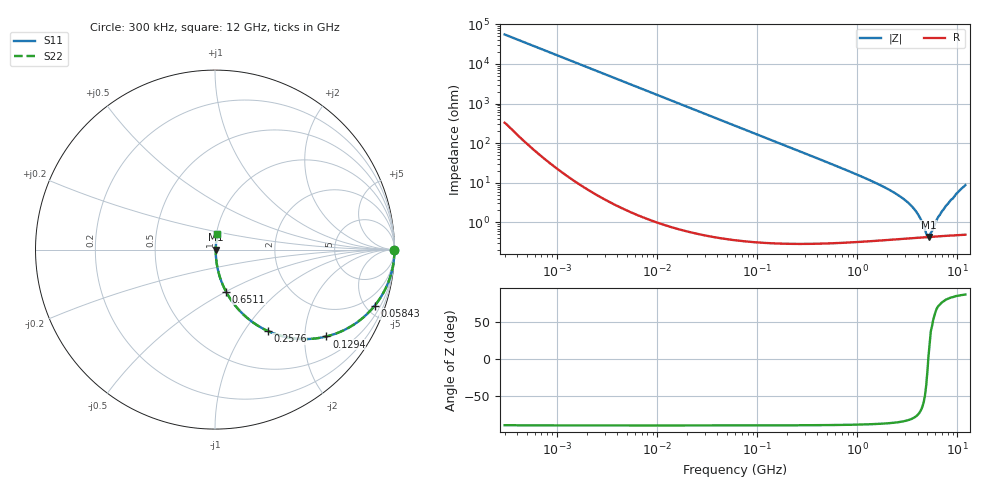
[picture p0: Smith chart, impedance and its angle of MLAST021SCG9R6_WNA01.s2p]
! MLAST021SCG9R6_WNA01  S-PARAMETER MODEL  ( General Type )
! Model Generated by TAIYO YUDEN Corporation (http://www.ty-top.com)
! Version 1.0
! TAIYO YUDEN Control No. 220901
! Copyright(c) 2022 TAIYO YUDEN CO.,LTD. All Rights Reserved.
! Product Description (link to TY-COMPAS)
! https://ds.yuden.co.jp/TYCOMPAS/or/detail?pn=MLAST021SCG9R6CWNA01&u=M
! Products Name : Multilayer Ceramic Capacitors
! Characteristics :
!  Capacitance : 9.6 pF , Rated Voltage : 25V , TCC : CG / C0G
!  Case Size : 0.25 x 0.125 / 0.0098 x 0.0049 [mm/inch] , Thickness : 0.125 / 0.0049 [mm/inch]
!  (Conditions: Temperature = 25 degC , DC Bias Current/Voltage = 0A / 0V)
! External Node Assignments :
!  1  o---| |---o  2
! GND o---------o GND
! Frequency Range : 0.3MHz  -  12000MHz  [ 401 STEP ]
# MHz S RI R 50
! Freq[MHz].  S11 Real  S11 Imag  S21 Real  S21 Imag  S12 Real  S12 Imag  S22 Real  S22 Imag
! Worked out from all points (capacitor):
!   401 points, 300 kHz to 12 GHz, reference 50 ohm
!   read as one part in series: C = 9.6 pF near 316.3 kHz
!   lowest |Z| = 428 mohm at 5.141 GHz (marker M1)
!   series resonance near 5.116 GHz, so ESL is about 100 pH
!   S11 on the Smith chart (normalised r, x): 300 kHz: open; 58.43 MHz: 1.01, -5.67; 129.4 MHz: 1.01, -2.56; 257.6 MHz: 1.01, -1.28; 651.1 MHz: 1.01, -0.50; 12 GHz: 1.01, +0.17
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0.3  1 -0.00181  1.4e-05 0.00181  1.4e-05 0.00181  1 -0.00181
1.769972  0.9999 -0.0107  0.000123 0.0107  0.000123 0.0107  0.9999 -0.0107
10.44266  0.996 -0.0627  0.00399 0.0627  0.00399 0.0627  0.996 -0.0627
25.70316  0.9764 -0.1514  0.0236 0.1514  0.0236 0.1514  0.9764 -0.1514
58.43137  0.8892 -0.3133  0.1108 0.3133  0.1108 0.3133  0.8892 -0.3133
60  0.8838 -0.3198  0.1162 0.3198  0.1162 0.3198  0.8838 -0.3198
129.3602  0.621 -0.484  0.379 0.484  0.379 0.484  0.621 -0.484
182.544  0.4515 -0.4961  0.5485 0.4961  0.5485 0.4961  0.4515 -0.4961
257.5933  0.2927 -0.4528  0.7073 0.4528  0.7073 0.4528  0.2927 -0.4528
353.9943  0.18 -0.3811  0.82 0.3811  0.82 0.3811  0.18 -0.3811
651.0506  0.0615 -0.2344  0.9385 0.2344  0.9385 0.2344  0.0615 -0.2344
2088.533  0.00791 -0.0654  0.9921 0.0654  0.9921 0.0654  0.00791 -0.0654
2870.14  0.00536 -0.0392  0.9946 0.0392  0.9946 0.0392  0.00536 -0.0392
3642.919  0.00449 -0.0222  0.9955 0.0222  0.9955 0.0222  0.00449 -0.0222
4158.869  0.00427 -0.0133  0.9957 0.0133  0.9957 0.0133  0.00427 -0.0133
4875.354  0.00422 -0.00301  0.9958 0.00301  0.9958 0.00301  0.00422 -0.00301
5140.631  0.00425 0.000295  0.9957 -0.000295  0.9957 -0.000295  0.00425 0.000295
5420.343  0.0043 0.00326  0.9957 -0.00326  0.9957 -0.00326  0.0043 0.00326
6354.153  0.00456 0.0122  0.9954 -0.0122  0.9954 -0.0122  0.00456 0.0122
7448.838  0.00505 0.0227  0.995 -0.0227  0.995 -0.0227  0.00505 0.0227
10236.47  0.00825 0.0589  0.9917 -0.0589  0.9917 -0.0589  0.00825 0.0589
12000  0.0122 0.0854  0.9878 -0.0854  0.9878 -0.0854  0.0122 0.0854
